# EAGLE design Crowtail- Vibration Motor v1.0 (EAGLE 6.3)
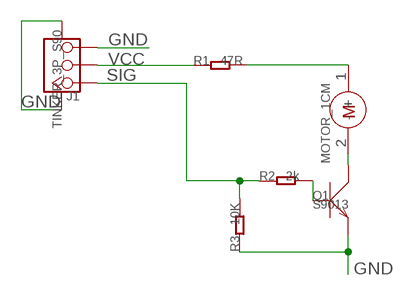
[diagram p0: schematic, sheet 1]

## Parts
J1  TINKER_3P_S90  [TINKER_3P_S90]
M1  MOTOR_1CM  [MOTOR_1CM]
Q1  S9013  TRANSISTOR-NPN-SOT23  [SOT23]
R1  47R  R-0603  [R0603]
R2  2k  R-0603  [R0603]
R3  10K  R-0603  [R0603]

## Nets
GND: J1.3 J1.SS1 J1.SS2 Q1.2(E) R3.1
N$1: Q1.1(B) R2.2
N$2: M1.1(+) R1.2
N$3: M1.2(-) Q1.3(C)
SIG: J1.1 R2.1 R3.2
VCC: J1.2 R1.1

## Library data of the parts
J1 = Connector:TINKER_3P_S90
M1 = EXT_moudle:MOTOR_1CM
Q1 = Discrete:TRANSISTOR-NPN*: NPN audion
R1-R3 = Discrete:R*

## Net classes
0 default: width 0.152 mm, drill 0.305 mm, clearance 0.152 mm

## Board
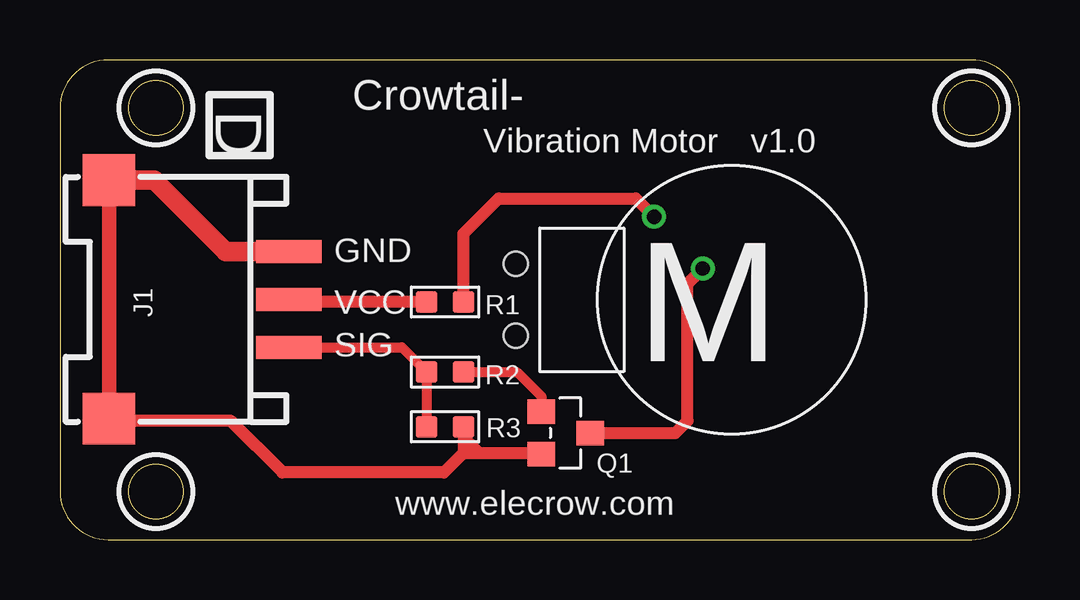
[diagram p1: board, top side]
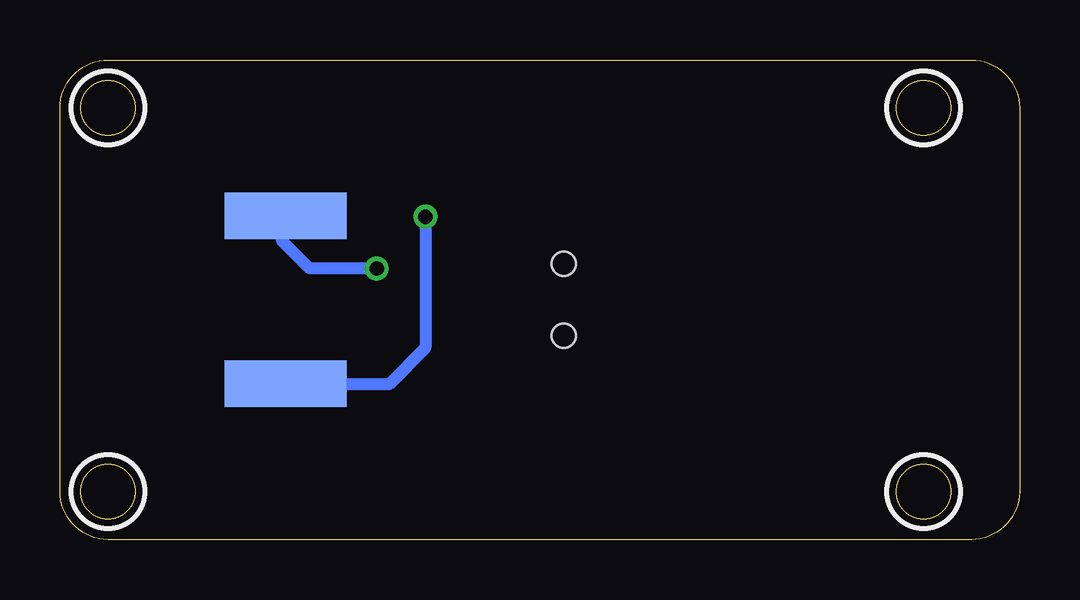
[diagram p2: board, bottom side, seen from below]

Size 40 x 20 mm. Coordinates in mm from the lower left corner, seen from the top.
Outline: 0,18 0,2 arc90 2,0 38,0 arc90 40,2 40,18 arc90 38,20 2,20 arc90 0,18
Outline: circle at 4,18 radius 1.14
Outline: circle at 4,2 radius 1.14
Outline: circle at 38,18 radius 1.14
Outline: circle at 38,2 radius 1.14
Copper layers (1*16): Top 0.035mm / dielectric 1.5mm / Bottom 0.035mm
Design rules "default *": minimum track width 10mil, minimum drill 24mil, track to track 8mil, track to pad 8mil, pad to pad 8mil, via to via 8mil, smd to smd 8mil, copper to edge 40mil, drill to drill 8mil, minimum pad ring 10mil, minimum via ring 8mil, stop-mask expansion 2mil, vias tented up to drill 100mil, thermal gap 10mil
tRestrict: area 2.5,16.5 to 5.5,19.5; area 2.5,0.5 to 5.5,3.5; area 36.5,16.5 to 39.5,19.5; area 36.5,0.5 to 39.5,3.5
bRestrict: area 2.5,16.5 to 5.5,19.5; area 2.5,0.5 to 5.5,3.5; area 36.5,16.5 to 39.5,19.5; area 36.5,0.5 to 39.5,3.5

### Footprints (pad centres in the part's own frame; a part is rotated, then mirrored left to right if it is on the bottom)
TINKER_3P_S90 = smd 0.965 x 2.74: 1 -1.984,-4.545; 2 0.016,-4.545; 3 2.016,-4.545 | smd 2.159 x 2.184: SS1 -4.958,2.955; SS2 4.99,2.955
MOTOR_1CM = smd 5.08 x 1.93 bottom: 1 -2.595,3.5; 2 -2.595,-3.5 | hole 1: 9,1.5; 9,-1.5
SOT23 = smd 1.016 x 1.143: 1 -0.889,-1.016; 2 0.889,-1.016; 3 0,1.016
R0603 = smd 0.889 x 0.889: 1 -0.762,0; 2 0.762,0

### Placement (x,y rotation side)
J1  5,10 90 top
M1  28,10 180 top
Q1  21.08,4.45 270 top
R1  16.05,9.91 0 top
R2  16.05,6.99 0 top
R3  16.05,4.7 180 top

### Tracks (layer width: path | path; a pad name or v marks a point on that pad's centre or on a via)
GND
  Top 0.508: 16.82,3.61 16,2.79 9.27,2.79 7.11,4.95 2.13,4.95 J1.SS1 | 16.82,3.61 20.02,3.61 Q1.2 | R3.1 16.82,3.61
  Top 0.61: J1.SS2 J1.SS1
  Top 0.813: J1.SS2 3.94,14.99 6.91,12.02 J1.3
N$1
  Top 0.406: R2.2 19.05,6.99 20.07,5.97 Q1.1
N$2  (via drill 0.6)
  Top 0.508: v24.77,13.46 24,14.22 18.29,14.22 16.82,12.75 R1.2
  Bottom 0.508: v24.77,13.46 24.77,8 26.29,6.48 30.57,6.48 M1.1
N$3  (via drill 0.6)
  Top 0.508: Q1.3 25.65,4.45 26.16,4.95 26.16,10.67 v26.8,11.3
  Bottom 0.508: v26.8,11.3 29.59,11.3 30.73,12.45 30.73,13.36 M1.2
N$4
  Top 0.508: 16.89,4.19 17.4,3.68
SIG
  Top 0.406: J1.1 14.26,8.02 R2.1 R3.2
VCC
  Top 0.508: R1.1 9.65,9.91 J1.2

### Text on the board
tPlace: D | Crowtail- | Vibration Motor | v1.0 | GND | VCC | SIG | www.elecrow.com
